(* Logix 5000 AddOnInstructionDefinition export AMP_Status_Code; software revision 20.04 *)

ADD_ON_INSTRUCTION AMP_Status_Code   (* revision 1.0 *)
// Applied Motion - Status Code AOI
// Help:
// The Status Code AOI uses the raw data stored in the Status Code word (Element 0 from Input Assembly 0x65) to set individual appropriately named boolean outputs.
VAR_INPUT
   Input : DINT; {required}   // Element 0 from Drive Input Assembly (0x65)
END_VAR
VAR_OUTPUT
   Motor_Enabled : BOOL; {access Read Only, visible}
   Sampling : BOOL; {access Read Only, visible}
   Drive_Fault : BOOL; {access Read Only, visible}
   In_Position : BOOL; {access Read Only, visible}
   Moving : BOOL; {access Read Only, visible}
   Jogging : BOOL; {access Read Only, visible}
   Stopping : BOOL; {access Read Only, visible}
   Waiting : BOOL; {access Read Only, visible}
   Saving : BOOL; {access Read Only, visible}
   Alarm_Present : BOOL; {access Read Only, visible}
   Homing : BOOL; {access Read Only, visible}
   Wait_Time : BOOL; {access Read Only, visible}
   Wizard_Running : BOOL; {access Read Only, visible}
   Checking_Encoder : BOOL; {access Read Only, visible}
   Q_Program_Running : BOOL; {access Read Only, visible}
   Initializing : BOOL; {access Read Only, visible}
END_VAR

ROUTINE Logic   (* ladder *)
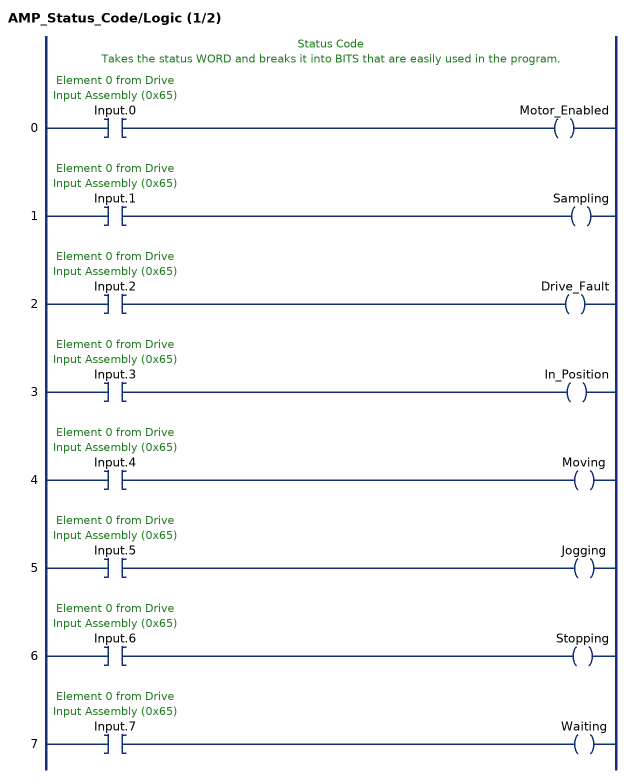
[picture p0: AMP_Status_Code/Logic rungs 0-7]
   // Status Code
   // Takes the status WORD and breaks it into BITS that are easily used in the program.
   0: XIC(Input.0)OTE(Motor_Enabled);
   1: XIC(Input.1)OTE(Sampling);
   2: XIC(Input.2)OTE(Drive_Fault);
   3: XIC(Input.3)OTE(In_Position);
   4: XIC(Input.4)OTE(Moving);
   5: XIC(Input.5)OTE(Jogging);
   6: XIC(Input.6)OTE(Stopping);
   7: XIC(Input.7)OTE(Waiting);
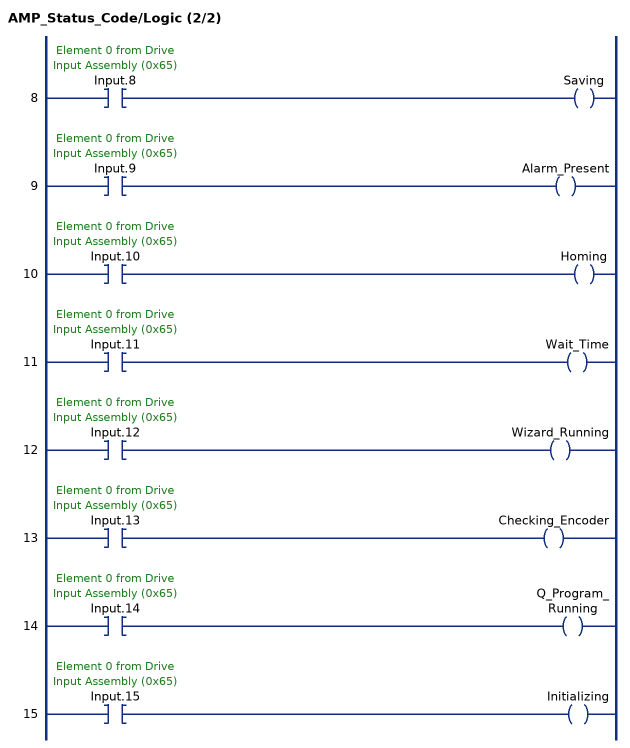
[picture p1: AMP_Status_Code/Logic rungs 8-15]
   8: XIC(Input.8)OTE(Saving);
   9: XIC(Input.9)OTE(Alarm_Present);
   10: XIC(Input.10)OTE(Homing);
   11: XIC(Input.11)OTE(Wait_Time);
   12: XIC(Input.12)OTE(Wizard_Running);
   13: XIC(Input.13)OTE(Checking_Encoder);
   14: XIC(Input.14)OTE(Q_Program_Running);
   15: XIC(Input.15)OTE(Initializing);
END_ROUTINE
END_ADD_ON_INSTRUCTION
